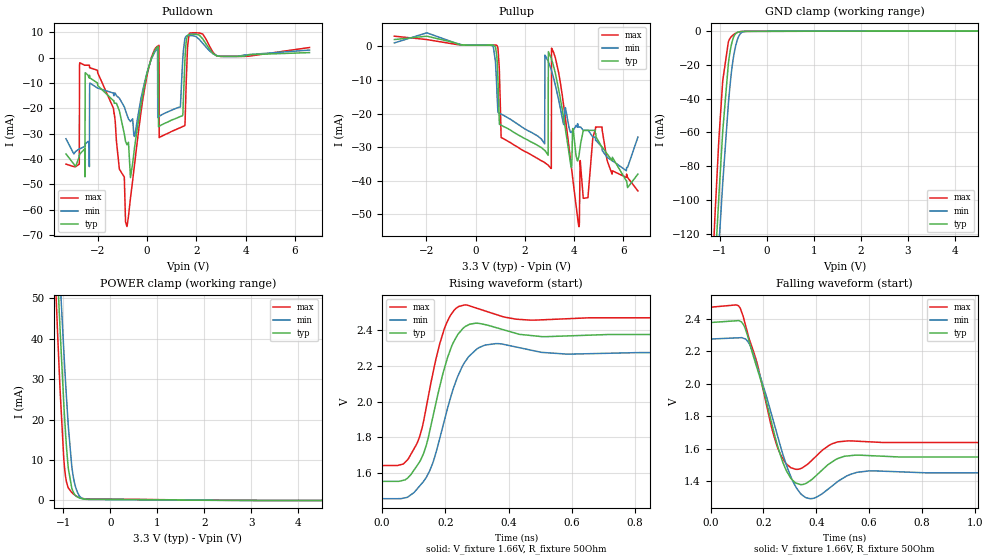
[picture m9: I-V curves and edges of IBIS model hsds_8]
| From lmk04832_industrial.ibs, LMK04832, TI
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|   hsds_8 Model
[Model]   hsds_8
Model_type   3-state
Polarity   Non-Inverting
Vmeas = 2.1
Vref = 1.66
Cref = 1pF
Rref = 50
|   typ   min   max
C_comp   2.136pF   2.117pF   2.176pF
|  Where Nom  PVT is Nominal Process,   3.3V,  25C
|   Fast PVT is Strong Process,   3.45V, -40C
|   Slow PVT is Weak Process,   3.15V, 85C
[Voltage Range]   3.3   3.15   3.45
|Junction Temperature
[Temperature Range]   25   85   -40
[Pullup Reference]   3.3   3.15   3.45
[Pulldown Reference]   0   0   0
[Power Clamp Reference]   3.3   3.15   3.45
[GND Clamp Reference]   0   0   0
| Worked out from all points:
|   GND clamp passes 1 mA (typ) near -0.64 V on its own axis
|   POWER clamp passes 1 mA (typ) near -0.71 V on its own axis
|   falling waveform, V_fixture 1.66V, R_fixture 50Ohm: 20-80 % time 83ps typ, 88.4ps min, 79.1ps max; typ from 2.38 V to 1.55 V
|   rising waveform, V_fixture 1.66V, R_fixture 50Ohm: 20-80 % time 68.2ps typ, 80.5ps min, 60ps max; typ from 1.55 V to 2.38 V
[Pulldown]
|   Voltage   I(typ)   I(min)   I(max)
-3.3V     -38mA      -32mA      -42mA
-2.76V    -39mA      -36mA      -42mA
-2.74V    -38mA      -36mA      -2mA
-2.53V    -47mA      -34mA      -3mA
-2.52V    -6mA       -35mA      -3mA
-820mV    -34.4mA    -22.6mA    -66.64mA
350mV     3.496mA    2.911mA    3.861mA
480mV     -27.06mA   -23.28mA   4.865mA
490mV     -27.06mA   -23.18mA   -31.55mA
1.53V     -1.89mA    7.312mA    -26.8mA
1.73V     9.246mA    8.692mA    9.689mA
6.6V      2mA        3mA        4mA
[GND Clamp]
|   Voltage   I(typ)   I(min)   I(max)
-3.3V     -1.535A    -1.479A    -1.61A
-1.52V    -370mA     -382mA     -361mA
-1.1V     -137mA     -164mA     -106mA
-1.09V    -132mA     -159mA     -101mA
-1.03V    -102mA     -131mA     -68.1mA
-1.02V    -96.6mA    -126mA     -63mA
-940mV    -59.2mA    -89.9mA    -29.3mA
-800mV    -15mA      -36.6mA    -5.02mA
-720mV    -4.43mA    -16.9mA    -2.35mA
-620mV    -719uA     -4.45mA    -754uA
-400mV    -186uA     -179uA     -203uA
6.6V      0A         0A         0A
[Pullup]
|   Voltage   I(typ)   I(min)   I(max)
-3.3V     2mA        1mA        3mA
870mV     -3.551mA   -13.46mA   243uA
1.04V     -23.47mA   -20.14mA   -27.11mA
2.81V     -30.92mA   -29.02mA   -34.53mA
2.82V     -31.02mA   -2.636mA   -34.63mA
2.95V     -32.42mA   -4.399mA   -35.33mA
2.96V     -1.587mA   -4.569mA   -35.43mA
3.07V     -3.452mA   -6.804mA   -36.32mA
3.09V     -3.87mA    -7.283mA   -556.9uA
4.2V      -32.7mA    -24mA      -53.58mA
4.88V     -26mA      -28mA      -24mA
6.6V      -38mA      -27mA      -43mA
[POWER Clamp]
|   Voltage   I(typ)   I(min)   I(max)
-3.3V     674mA      627mA      733mA
-1.17V    68.5mA     78.7mA     55.6mA
-1.12V    55.5mA     66.8mA     41.4mA
-1.07V    43mA       55.2mA     28mA
-980mV    22.3mA     35.4mA     9.16mA
-950mV    16.5mA     29.2mA     5.87mA
-890mV    7.82mA     18.1mA     3.07mA
-800mV    2.46mA     6.88mA     1.77mA
-740mV    1.26mA     3.45mA     1.23mA
-670mV    705uA      1.4mA      773uA
-410mV    296uA      245uA      367uA
6.6V      0A         0A         0A
[Ramp]
R_load = 50
|   typ   min   max
dV/dt_r   0.494275/6.78608e-11   0.491758/8.00315e-11   0.497238/5.98217e-11
dV/dt_f   0.494242/8.30006e-11   0.491736/8.81455e-11   0.497195/7.91505e-11
[Falling Waveform]
V_fixture = 1.66V
V_fixture_min = 1.51V
V_fixture_max = 1.81V
R_fixture = 50Ohm
C_fixture = 0F
|   Time   V(typ)   V(min)   V(max)
0s        2.376V     2.274V     2.469V
105.6ps   2.387V     2.282V     2.478V
144.1ps   2.272V     2.252V     2.287V
177.3ps   2.089V     2.102V     2.119V
252ps     1.627V     1.689V     1.615V
288.5ps   1.461V     1.494V     1.505V
323.7ps   1.389V     1.364V     1.474V
385.4ps   1.415V     1.295V     1.533V
521ps     1.557V     1.438V     1.649V
20ns      1.552V     1.454V     1.641V
[Rising Waveform]
V_fixture = 1.66V
V_fixture_min = 1.51V
V_fixture_max = 1.81V
R_fixture = 50Ohm
C_fixture = 0F
|   Time   V(typ)   V(min)   V(max)
0s        1.552V     1.455V     1.641V
80ps      1.57V      1.463V     1.672V
119ps     1.664V     1.527V     1.806V
139ps     1.752V     1.573V     1.964V
198.8ps   2.199V     1.908V     2.42V
224.9ps   2.331V     2.072V     2.506V
261.2ps   2.419V     2.221V     2.543V
359.9ps   2.415V     2.326V     2.489V
584ps     2.368V     2.266V     2.465V
20ns      2.376V     2.274V     2.469V
